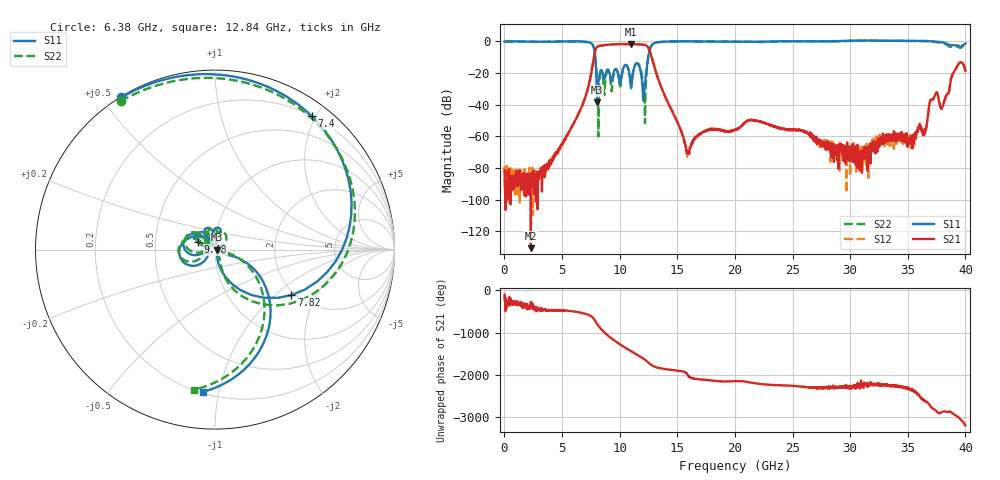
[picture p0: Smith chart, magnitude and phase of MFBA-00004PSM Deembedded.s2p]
!Keysight Technologies,N5247B,US58420632,A.15.75.19
!Date: Thursday, September 22, 2022 11:14:40
!Correction: S11(C  2-Port  )
!S41(C  2-Port  )
!S14(C  2-Port  )
!S44(C  2-Port  )
!S2P File: Measurements: S11, S41, S14, S44:
# Hz S  dB  R 50
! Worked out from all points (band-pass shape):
!   2000 points, 20 MHz to 40 GHz, reference 50 ohm
!   highest |S21| = -1.68 dB at 11 GHz (marker M1); lowest = -130.9 dB at 2.3 GHz (marker M2)
!   |S21| within 3 dB of the highest: 7.937 GHz to 12.54 GHz (4.602 GHz wide, 44.9 % of centre)
!   lowest |S11| = -38.6 dB at 8.04 GHz (marker M3), VSWR 1.02, Z = 51.2 - j0.0962 ohm
!   |S11| at or under -10 dB: 7.882 GHz to 12.48 GHz (4.595 GHz wide, 45.1 % of centre)
!   |S22| runs from -60.1 to 0.4 dB; largest |S21 - S12| = 0.0011
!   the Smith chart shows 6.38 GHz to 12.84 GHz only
!   S11 on the Smith chart (normalised r, x): 6.38 GHz: 0.00, +0.56; 7.4 GHz: 0.20, +1.94; 7.82 GHz: 1.92, -1.29; 9.48 GHz: 0.83, +0.07; 12.84 GHz: 0.21, -0.90
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2e7  -0.16 -0.9  -81.36 -96.7  -78.96 -150.9  -0.11 -0.9
2.3e9  -0.20 -93.3  -130.89 89.3  -97.82 -17.5  -0.35 -93.8
6.38e9  -0.04 121.7  -46.66 -154.9  -46.60 -154.5  -0.18 122.5
6.7e9  -0.11 105.4  -41.61 -172.0  -41.57 -171.8  -0.29 105.2
7.4e9  -0.74 54.1  -25.14 126.9  -25.14 126.9  -0.91 49.0
7.82e9  -6.09 -30.7  -7.85 23.0  -7.85 23.0  -5.80 -36.2
8.04e9  -38.62 -4.6  -3.62 -75.5  -3.62 -75.5  -23.37 -65.3
8.68e9  -24.16 104.5  -2.35 82.4  -2.35 82.4  -33.96 99.2
9.06e9  -18.63 100.7  -2.12 -9.5  -2.12 -9.6  -19.40 85.1
9.48e9  -19.71 155.0  -1.92 -98.9  -1.92 -98.9  -21.03 158.3
1.036e10  -16.11 -174.7  -1.79 100.2  -1.79 100.1  -16.49 178.6
1.1e10  -29.67 -176.9  -1.68 -4.5  -1.68 -4.5  -25.99 170.7
1.152e10  -13.97 -175.8  -1.94 -88.2  -1.94 -88.2  -13.82 -178.7
1.2e10  -30.59 102.1  -2.04 -169.7  -2.04 -169.7  -24.20 153.0
1.284e10  -1.99 -94.7  -11.59 11.1  -11.59 11.1  -2.06 -98.5
1.336e10  -0.54 -141.1  -24.09 -40.5  -24.09 -40.6  -0.60 -142.1
1.588e10  -0.02 147.8  -70.72 157.4  -70.32 159.9  -0.07 150.6
2.002e10  -0.30 60.9  -55.80 0.8  -56.14 2.2  -0.19 61.5
2.668e10  -0.05 -15.4  -59.63 -145.4  -60.65 -148.2  -0.00 -16.6
3.334e10  0.37 -7.7  -60.91 -104.7  -60.40 -78.6  0.27 -15.3
3.644e10  0.25 -2.2  -58.38 -106.5  -58.38 -102.1  0.13 -1.3
4e10  -1.48 -15.8  -18.67 28.9  -18.66 28.9  -1.98 -29.2
